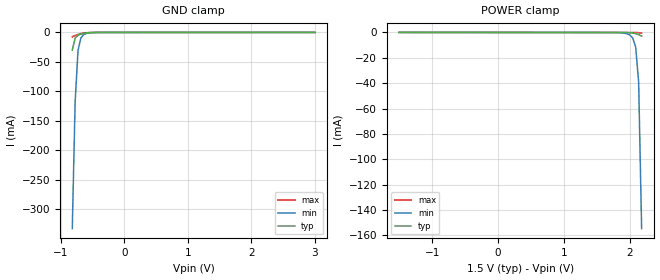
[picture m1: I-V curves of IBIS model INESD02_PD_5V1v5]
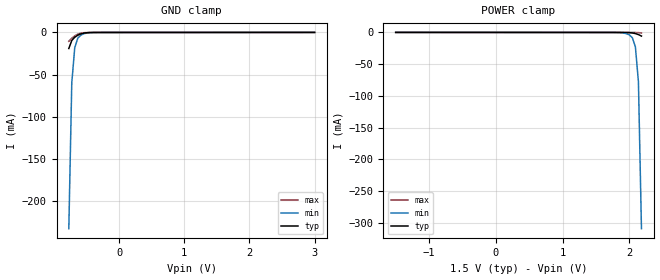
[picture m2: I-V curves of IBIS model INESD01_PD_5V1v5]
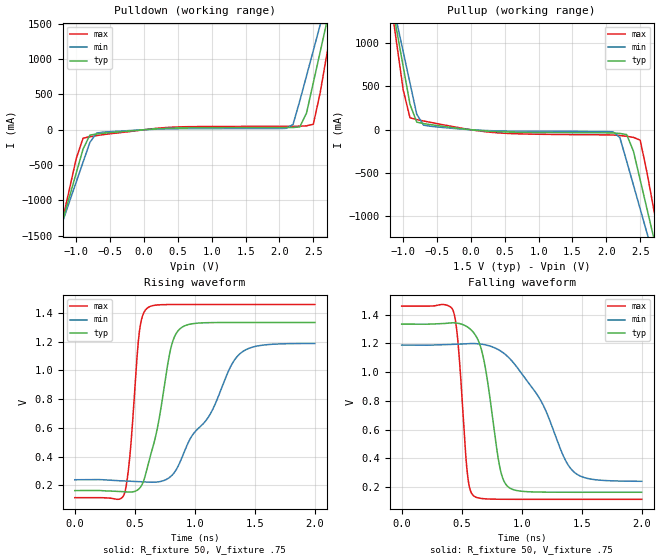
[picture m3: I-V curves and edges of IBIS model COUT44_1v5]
|   This file is an IBIS representation of the   |
|   Integrated Devices Technology , Inc.   |
|   ICS830154-09   |
|   OVER-VOLTAGE 1.5V TOLERANT, 1:4 FANOUT BUFFER   |
[IBIS Ver]   4.1
[File name]   830154_09.ibs
[File Rev]   1.0
[Date]   18 Aug 2010
[Source]   Originated at Integrated Device Technology, Inc.
[Disclaimer]
IDT hereby grants the user of this IBIS model a non-exclusive,
nontransferable license to use this IBIS model under the following terms.
Before using this IBIS model, the user should read this license.
If the user does not accept these terms,  the IBIS model should be
returned to IDT within 30 days.
   The user is granted this license only to use the IBIS model and
is not granted rights to sell, load, rent, lease or license the IBIS
model in whole or in part, or in modified form to anyone other than
user. User may modify the IBIS model to suit its specific
applications but rights to derivative works and such modifications
shall belong to IDT.
   This IBIS model is provided on an "AS IS" basis and IDT makes
absolutely no warranty with respect to the information contained
herein. IDT DISCLAIMS AND CUSTOMER WAIVES ALL WARRANTIES, EXPRESS
OR IMPLIED, INCLUDING WARRANTIES OF MERCHANTABILITY OR FITNESS FOR
A PARTICULAR PURPOSE. The entire risk as to quality and performance
is with the Customer. ACCORDINGLY, IN NO EVENT SHALL THE COMPANY BE
LIABLE FOR ANY DAMAGES, WHETHER IN CONTRACT OR TORT,INCLUDING ANY
LOST PROFITS OR OTHER INCIDENTAL, CONSEQUENTIAL, EXEMPLARY, OR
PUNITIVE DAMAGES ARISING OUT OF THE USE OR APPLICATION OF THE IBIS
model provided in this package. Further, IDT reserves the right to
make changes without notice to any product herein to improve
reliability, function, or design. IDT does not convey any license
under patent rights or any other intellectual property rights,
including those of third parties.
   IDT is not obligated to provide maintenance or support
for the licensed IBIS model.
[Copyright]   Copyright 2010 by Integrated Device Technology, Inc.
[Component]   830154G_08
[Manufacturer] Integrated Device Technology, Inc.
[Package]
|TSSOP 8 Lead
|   typ   min   max
R_pkg   52.5m   48.8m   56.2m
L_pkg   1.381nH   1.275nH   1.486nH
C_pkg   0.236pF   0.230pF   0.242pF
[Pin]   signal_name   model_name   R_pin   L_pin   C_pin
1   CLK_IN   INESD02_PD_5Vr   56.2m   1.486n   0.242p
2   VDD   POWER   48.8m   1.275n   0.230p
3   nOE   INESD01_PD_5Vr   48.8m   1.275n   0.230p
4   GND   GND   56.2m   1.468n   0.242p
5   Q3   COUT44   56.2m   1.486n   0.242p
6   Q2   COUT44   48.8m   1.275n   0.230p
7   Q1   COUT44   48.8m   1.275n   0.230p
8   Q4   COUT44   56.2m   1.468n   0.242p
[Component]   830154M_08
[Manufacturer] Integrated Device Technology, Inc.
[Package]
|SOIC 8 Lead
|   typ   min   max
R_pkg   57.05m   55.5m   58.6m
L_pkg   1.769nH   1.570nH   1.968nH
C_pkg   0.269pF   0.252pF   0.286pF
[Pin]   signal_name   model_name   R_pin   L_pin   C_pin
1   CLK_IN   INESD02_PD_5Vr   58.6m   1.968n   0.286p
2   VDD   POWER   55.5m   1.570n   0.252p
3   nOE   INESD01_PD_5Vr   55.5m   1.570n   0.252p
4   GND   GND   56.6m   1.968n   0.286p
5   Q3   COUT44   58.6m   1.968n   0.286p
6   Q2   COUT44   55.5m   1.570n   0.252p
7   Q1   COUT44   55.5m   1.570n   0.252p
8   Q4   COUT44   56.6m   1.968n   0.286p
[Model Selector] INESD02_PD_5Vr
INESD02_PD_5V1v5  Buffer selection for 1v5
INESD02_PD_5V1v8  Buffer selection for 1v8
[Model Selector] INESD01_PD_5Vr
INESD01_PD_5V1v5  Buffer selection for 1v5
INESD01_PD_5V1v8  Buffer selection for 1v8
[Model Selector] COUT44
COUT44_1v5  Buffer selection for 1v5
COUT44_1v8  Buffer selection for 1v8
| Models and submodels in the file (6): INESD02_PD_5V1v5 (Input), INESD01_PD_5V1v5 (Input), COUT44_1v5 (Output), INESD02_PD_5V1v8 (Input), INESD01_PD_5V1v8 (Input), COUT44_1v8 (Output)
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[Model] INESD02_PD_5V1v5
Model_type   Input
Polarity   Non-Inverting
Vinl = 0.49V
Vinh = 1.04V
|   typ   min   max
C_comp   2pF   1.5pF   2.5pF
|   typ   min   max
[Voltage range]   1.5V   1.4V   1.6V
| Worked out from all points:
|   GND clamp passes 1 mA (typ) near -0.60 V on its own axis
[GND_clamp]
|Voltage   I (typ)   I (min)   I (max)
|Note, modeling breaks down at 250mA and above.  This is well beyond the functional   |
|operating range of the device.  Should this scenario occur, catastrophic failure and   |
|possible damage to the device and/or board is of higher concern than the I-V curve   |
|behavior.  The IBIS checker will flag currents in excess of 10A with warnings.  Lines   |
|with currents in excess of 0.35 A have been commented out.  The points still remain|
|available to the user if the user desires to use them.   |
|-1.50000e+00   -3.89380e+00   -3.68384e+00   -4.28297e+00
|-1.45455e+00   -3.62541e+00   -3.46019e+00   -3.94026e+00
|-1.40909e+00   -3.35704e+00   -3.23656e+00   -3.59755e+00
|-1.36364e+00   -3.08869e+00   -3.01295e+00   -3.25485e+00
|-1.31818e+00   -2.82035e+00   -2.78937e+00   -2.91216e+00
|-1.27273e+00   -2.55204e+00   -2.56581e+00   -2.56949e+00
|-1.22727e+00   -2.28376e+00   -2.34228e+00   -2.22683e+00
|-1.18182e+00   -2.01551e+00   -2.11879e+00   -1.88421e+00
|-1.13636e+00   -1.74730e+00   -1.89534e+00   -1.54161e+00
|-1.09091e+00   -1.47913e+00   -1.67194e+00   -1.19905e+00
|-1.04545e+00   -1.21102e+00   -1.44858e+00   -8.56537e-01
|-1.00000e+00   -9.42966e-01   -1.22529e+00   -5.14085e-01
|-9.54545e-01   -6.74990e-01   -1.00206e+00   -1.71708e-01
|-9.09091e-01   -4.07111e-01   -7.78918e-01   -2.82167e-02
|-8.63636e-01   -1.40646e-01   -5.55864e-01   -1.11530e-02
-818.2mV  -29.87mA   -332.9mA   -7.406mA
-772.7mV  -9.527mA   -116.5mA   -5.226mA
-727.3mV  -4.766mA   -29.91mA   -3.451mA
-681.8mV  -2.863mA   -9.094mA   -2.032mA
-636.4mV  -1.688mA   -3.525mA   -1.028mA
-545.5mV  -426uA     -809.3uA   -164.8uA
-409.1mV  -28.71uA   -73.49uA   -9.493uA
3V        58.45uA    73.09uA    45.29uA
[Power_clamp]
|Voltage   I (typ)   I (min)   I (max)
|Note, modeling breaks down at 250mA and above.  This is well beyond the functional   |
|operating range of the device.  Should this scenario occur, catastrophic failure and   |
|possible damage to the device and/or board is of higher concern than the I-V curve   |
|behavior.  The IBIS checker will flag currents in excess of 10A with warnings.  Lines   |
|with currents in excess of 0.35 A have been commented out.  The points still remain|
|available to the user if the user desires to use them.   |
-1.5V     58.45uA    70.65uA    46.8uA
1.773V    -5.708uA   -37.98uA   -2.608uA
1.909V    -28.71uA   -446.9uA   -4.741uA
2V        -180.1uA   -1.901mA   -8.464uA
2.045V    -426uA     -4.182mA   -17.48uA
2.091V    -902.2uA   -11.33mA   -46.97uA
2.136V    -1.688mA   -38.87mA   -134.1uA
2.182V    -2.863mA   -154.7mA   -364.8uA
| 2.22727e+00   -4.76564e-03   -3.77495e-01   -8.79105e-04
| 2.27273e+00   -9.52685e-03   -6.00467e-01   -1.79677e-03
| 2.31818e+00   -2.98680e-02   -8.23539e-01   -3.13669e-03
| 2.36364e+00   -1.40646e-01   -1.04670e+00   -4.84434e-03
| 2.40909e+00   -4.07111e-01   -1.26994e+00   -6.91945e-03
| 2.45455e+00   -6.74990e-01   -1.49325e+00   -1.00747e-02
| 2.50000e+00   -9.42966e-01   -1.71661e+00   -2.17627e-02
| 2.54545e+00   -1.21102e+00   -1.94003e+00   -1.14024e-01
| 2.59091e+00   -1.47913e+00   -2.16349e+00   -4.45603e-01
| 2.63636e+00   -1.74730e+00   -2.38699e+00   -7.88042e-01
| 2.68182e+00   -2.01551e+00   -2.61052e+00   -1.13054e+00
| 2.72727e+00   -2.28376e+00   -2.83408e+00   -1.47309e+00
| 2.77273e+00   -2.55204e+00   -3.05767e+00   -1.81568e+00
| 2.81818e+00   -2.82035e+00   -3.28129e+00   -2.15831e+00
| 2.86364e+00   -3.08869e+00   -3.50492e+00   -2.50095e+00
| 2.90909e+00   -3.35704e+00   -3.72857e+00   -2.84362e+00
| 2.95455e+00   -3.62541e+00   -3.95224e+00   -3.18631e+00
| 3.00000e+00   -3.89380e+00   -4.17593e+00   -3.52901e+00
[Model] INESD01_PD_5V1v5
Model_type   Input
Polarity   Non-Inverting
Vinl = 0.49V
Vinh = 1.04V
|   typ   min   max
C_comp   2pF   1.5pF   2.5pF
|   typ   min   max
[Voltage range]   1.5V   1.4V   1.6V
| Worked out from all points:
|   GND clamp passes 1 mA (typ) near -0.55 V on its own axis
[GND_clamp]
|Voltage   I (typ)   I (min)   I (max)
|Note, modeling breaks down at 250mA and above.  This is well beyond the functional   |
|operating range of the device.  Should this scenario occur, catastrophic failure and   |
|possible damage to the device and/or board is of higher concern than the I-V curve   |
|behavior.  The IBIS checker will flag currents in excess of 10A with warnings.  Lines   |
|with currents in excess of 0.35 A have been commented out.  The points still remain|
|available to the user if the user desires to use them.   |
|-1.50000e+00   -7.78759e+00   -7.36766e+00   -8.56594e+00
|-1.45455e+00   -7.25081e+00   -6.92037e+00   -7.88051e+00
|-1.40909e+00   -6.71407e+00   -6.47311e+00   -7.19509e+00
|-1.36364e+00   -6.17736e+00   -6.02589e+00   -6.50969e+00
|-1.31818e+00   -5.64069e+00   -5.57872e+00   -5.82432e+00
|-1.27273e+00   -5.10407e+00   -5.13161e+00   -5.13897e+00
|-1.22727e+00   -4.56751e+00   -4.68455e+00   -4.45367e+00
|-1.18182e+00   -4.03101e+00   -4.23757e+00   -3.76841e+00
|-1.13636e+00   -3.49459e+00   -3.79067e+00   -3.08322e+00
|-1.09091e+00   -2.95826e+00   -3.34386e+00   -2.39810e+00
|-1.04545e+00   -2.42203e+00   -2.89715e+00   -1.71308e+00
|-1.00000e+00   -1.88593e+00   -2.45056e+00   -1.02817e+00
|-9.54545e-01   -1.34998e+00   -2.00411e+00   -3.43421e-01
|-9.09091e-01   -8.14221e-01   -1.55783e+00   -5.64379e-02
|-8.63636e-01   -2.81291e-01   -1.11172e+00   -2.23101e-02
|-8.18182e-01   -5.97340e-02   -6.65821e-01   -1.48150e-02
-772.7mV  -19.05mA   -233mA     -10.45mA
-727.3mV  -9.528mA   -59.82mA   -6.902mA
-681.8mV  -5.721mA   -18.18mA   -4.063mA
-636.4mV  -3.371mA   -7.042mA   -2.052mA
-590.9mV  -1.797mA   -3.283mA   -874.2uA
-500mV    -351.6uA   -755.3uA   -108.7uA
-363.6mV  -19.44uA   -56.15uA   -6.787uA
3V        58.45uA    73.09uA    45.29uA
[Power_clamp]
|Voltage   I (typ)   I (min)   I (max)
|Note, modeling breaks down at 250mA and above.  This is well beyond the functional   |
|operating range of the device.  Should this scenario occur, catastrophic failure and   |
|possible damage to the device and/or board is of higher concern than the I-V curve   |
|behavior.  The IBIS checker will flag currents in excess of 10A with warnings.  Lines   |
|with currents in excess of 0.35 A have been commented out.  The points still remain|
|available to the user if the user desires to use them.   |
-1.5V     58.45uA    70.65uA    46.8uA
1.773V    -6.106uA   -67.07uA   -2.608uA
1.909V    -49.61uA   -883.5uA   -4.817uA
2V        -351.6uA   -3.793mA   -10.91uA
2.045V    -843.7uA   -8.355mA   -28.33uA
2.091V    -1.797mA   -22.65mA   -86.86uA
2.136V    -3.371mA   -77.73mA   -261uA
2.182V    -5.721mA   -309.3mA   -723.2uA
| 2.22727e+00   -9.52796e-03   -7.54983e-01   -1.75373e-03
| 2.27273e+00   -1.90511e-02   -1.20093e+00   -3.59154e-03
| 2.31818e+00   -5.97340e-02   -1.64707e+00   -6.27371e-03
| 2.36364e+00   -2.81291e-01   -2.09339e+00   -9.69076e-03
| 2.40909e+00   -8.14221e-01   -2.53987e+00   -1.38422e-02
| 2.45455e+00   -1.34998e+00   -2.98649e+00   -2.01535e-02
| 2.50000e+00   -1.88593e+00   -3.43322e+00   -4.35298e-02
| 2.54545e+00   -2.42203e+00   -3.88005e+00   -2.28053e-01
| 2.59091e+00   -2.95826e+00   -4.32696e+00   -8.91210e-01
| 2.63636e+00   -3.49459e+00   -4.77396e+00   -1.57609e+00
| 2.68182e+00   -4.03101e+00   -5.22102e+00   -2.26109e+00
| 2.72727e+00   -4.56751e+00   -5.66815e+00   -2.94619e+00
| 2.77273e+00   -5.10407e+00   -6.11533e+00   -3.63137e+00
| 2.81818e+00   -5.64069e+00   -6.56256e+00   -4.31661e+00
| 2.86364e+00   -6.17736e+00   -7.00982e+00   -5.00191e+00
| 2.90909e+00   -6.71407e+00   -7.45713e+00   -5.68725e+00
| 2.95455e+00   -7.25081e+00   -7.90446e+00   -6.37262e+00
| 3.00000e+00   -7.78759e+00   -8.35183e+00   -7.05801e+00
[Model] COUT44_1v5
Model_type   Output
Polarity   Non-Inverting
Vmeas = .8
Rref = 50
Cref = 0
Vref = .75
|   typ   min   max
C_comp   2pF   1.5pF   2.5pF
|   typ   min   max
[Voltage range]  1.5V   1.425V   1.575V
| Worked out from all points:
|   slope of the pulldown table from 0 to 0.225 V, typ, clamps not added: 15 ohm
|   slope of the pullup table from 0 to 0.225 V, typ, clamps not added: 15.1 ohm
|   rising waveform, R_fixture 50, V_fixture .75: 20-80 % time 159ps typ, 372ps min, 71.5ps max; typ from 0.164 V to 1.33 V
|   falling waveform, R_fixture 50, V_fixture .75: 20-80 % time 124ps typ, 348ps min, 66.3ps max; typ from 1.33 V to 0.164 V
[pulldown]
|Voltage   I (typ)   I (min)   I (max)
-3.3V     -8.323A    -7.168A    -10.22A
-1.3V     -1.614A    -1.572A    -1.688A
-900mV    -271.8mA   -457.1mA   -119.5mA
-700mV    -59.3mA    -46.39mA   -82.97mA
2.1V      30.75mA    19.84mA    48.6mA
2.2V      31.86mA    73.93mA    49.02mA
2.4V      237.7mA    764.4mA    55.05mA
2.5V      666.9mA    1.121A     78.82mA
2.6V      1.097A     1.479A     517.4mA
2.7V      1.529A     1.838A     1.069A
2.8V      1.961A     2.196A     1.622A
6.6V      18.72A     16.1A      23.02A
[pullup]
|Voltage   I (typ)   I (min)   I (max)
-3.3V     10.79A     9.265A     13.29A
-1.2V     1.603A     1.626A     1.578A
-1.1V     1.166A     1.264A     1.019A
-900mV    294.2mA    540.3mA    138.3mA
-700mV    71.14mA    53.15mA    101mA
2.1V      -37.71mA   -24.67mA   -60.94mA
2.3V      -55.71mA   -363.8mA   -76.05mA
2.5V      -580.7mA   -915.6mA   -120.9mA
2.6V      -914.4mA   -1.193A    -492.4mA
2.7V      -1.249A    -1.47A     -919.4mA
2.8V      -1.583A    -1.748A    -1.347A
6.6V      -14.33A    -12.39A    -17.57A
[Ramp]
|   typ   min   max
dV/dt_r   .944/.233n   .853/.277n   1.04/.188n
dV/dt_f   .944/.199n   .853/.245n   1.04/.152n
[Rising Waveform]
R_fixture = 50
V_fixture = .75
V_fixture_max = .7875
V_fixture_min = .7125
C_fixture = 0.0p
| Time   typ   min   max
0s        163.8mV    239.2mV    114.8mV
411.6ps   155.6mV    230.9mV    139.1mV
459.9ps   153.3mV    229.3mV    415.3mV
537.6ps   178.5mV    226.1mV    1.267V
602.7ps   320.2mV    223mV      1.433V
690.9ps   611.4mV    223.8mV    1.456V
800.1ps   1.156V     262.8mV    1.459V
877.8ps   1.291V     364.9mV    1.459V
1.376ns   1.334V     1.116V     1.459V
1.999ns   1.334V     1.188V     1.459V
[Falling Waveform]
R_fixture = 50
V_fixture = .75
V_fixture_max = .7875
V_fixture_min = .7125
C_fixture = 0.0p
| Time   typ   min   max
0s        1.334V     1.188V     1.459V
430.5ps   1.343V     1.193V     1.423V
472.5ps   1.339V     1.194V     1.175V
548.1ps   1.314V     1.198V     287.5mV
600.6ps   1.273V     1.199V     138.1mV
678.3ps   1.109V     1.193V     119.4mV
812.7ps   357.6mV    1.153V     115.3mV
882ps     205.1mV    1.109V     115mV
1.43ns    163.9mV    308.6mV    114.8mV
1.999ns   163.8mV    240.2mV    114.8mV
